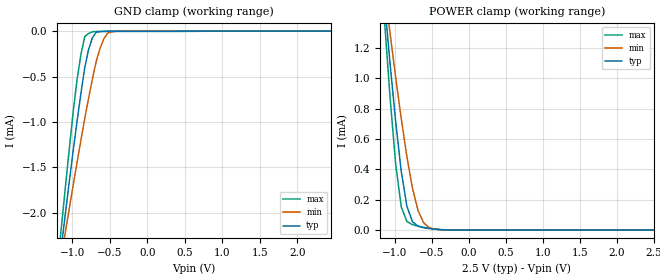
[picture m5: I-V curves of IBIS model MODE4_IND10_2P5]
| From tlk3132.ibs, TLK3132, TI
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|   Model Cell MODE4_IND10_2P5
|MODE4_IND10_2P5
[Model]   MODE4_IND10_2P5
Model_type   Input
Polarity   Non-Inverting
Vinl =  0.7V
Vinh =  1.7V
C_comp   0.5589689p   0.5140408p   0.6098818p
[Model Spec]
Vinl   0.7V   0.7V   0.7V
Vinh   1.7V   1.7V   1.7V
[Temperature Range]   25   125   -40
[Voltage Range]   2.5   2.375   2.625
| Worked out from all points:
|   GND clamp passes 1 mA (typ) near -0.94 V on its own axis
|   POWER clamp passes 1 mA (typ) near -1.04 V on its own axis
[POWER_clamp]
|   voltage   I(typ)   I(min)   I(max)
-2.5V     9.467mA    7.301mA    11.49mA
-1.136V   1.511mA    1.597mA    1.389mA
-1.111V   1.374mA    1.497mA    1.218mA
-1.061V   1.099mA    1.298mA    876.7uA
-984.8mV  715.3uA    1.008mA    436.5uA
-909.1mV  386.1uA    733.4uA    152.6uA
-833.3mV  157.5uA    484uA      56.45uA
-757.6mV  54.91uA    275.5uA    34.89uA
-681.8mV  24.34uA    127.4uA    25.24uA
-606.1mV  15.13uA    47.24uA    17.31uA
-454.5mV  5.622uA    4.961uA    5.593uA
2.5V      20.79nA    32.26nA    32.83nA
[GND_clamp]
|   voltage   I(typ)   I(min)   I(max)
-2.5V     -11.84mA   -9.505mA   -13.64mA
-1.187V   -2.664mA   -2.695mA   -2.515mA
-1.136V   -2.315mA   -2.439mA   -2.089mA
-1.086V   -1.972mA   -2.185mA   -1.673mA
-934.3mV  -984uA     -1.439mA   -527.1uA
-833.3mV  -402.6uA   -963.1uA   -60.65uA
-782.8mV  -205.6uA   -741.4uA   -26.89uA
-732.3mV  -75.89uA   -532.9uA   -8.115uA
-631.3mV  -6.376uA   -193.6uA   -4.083uA
-530.3mV  -1.911uA   -23.41uA   -3.92uA
-479.8mV  -1.865uA   -9.998uA   -3.899uA
2.449V    20.28nA    35.68nA    30.94nA
